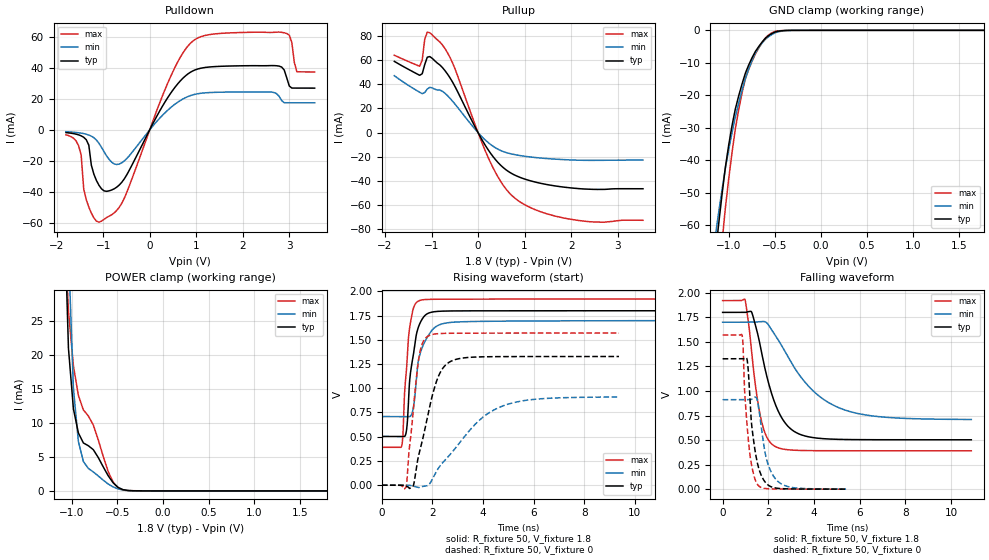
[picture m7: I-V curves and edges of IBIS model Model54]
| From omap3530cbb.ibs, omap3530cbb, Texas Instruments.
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| Model based on original model for CCPV2_7LM
|   Sub model CCPV2_7LM_SN
[model]   Model54
|[Input Load]   PI
|[Output Drive]
|Voltage   1.8V
|Mode   I/O
Model_type   I/O
Polarity   Non-Inverting
Enable   Active-Low
Vinl =  0.63
Vinh =  1.17
Cref =  15.0000pF
Rref =  100.0000M
Vref =  0V
Vmeas =  0.9
C_comp   5.837306p   5.73806p   5.865695p
[Model Spec]
Vinl   0.63   0.595   0.672
Vinh   1.17   1.105   1.248
[Temperature Range]   25   125   -40
[Voltage Range]   1.8   1.7   1.92
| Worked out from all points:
|   slope of the pulldown table from 0 to 0.27 V, typ, clamps not added: 17.9 ohm
|   slope of the pullup table from 0 to 0.27 V, typ, clamps not added: 15.8 ohm
|   GND clamp passes 1 mA (typ) near -0.53 V on its own axis
|   POWER clamp passes 1 mA (typ) near -0.53 V on its own axis
|   rising waveform, R_fixture 50, V_fixture 1.8: 20-80 % time 320ps typ, 436ps min, 234ps max; typ from 0.503 V to 1.8 V
|   rising waveform, R_fixture 50, V_fixture 0: 20-80 % time 728ps typ, 1.88ns min, 370ps max; typ from 0 V to 1.33 V
|   falling waveform, R_fixture 50, V_fixture 1.8: 20-80 % time 928ps typ, 1.98ns min, 523ps max; typ from 1.8 V to 0.503 V
|   falling waveform, R_fixture 50, V_fixture 0: 20-80 % time 361ps typ, 469ps min, 294ps max; typ from 1.33 V to 0 V
[POWER_clamp]
-1.8V     2.373A     2.073A     2.673A
-1.055V   29.19mA    52.52mA    31.79mA
-1.036V   21.01mA    35.61mA    26.49mA
-1.018V   18.03mA    28.77mA    23.8mA
-981.8mV  12.07mA    15.08mA    18.42mA
-927.3mV  8.532mA    7.272mA    14.05mA
-872.7mV  7.067mA    4.332mA    11.93mA
-818.2mV  6.655mA    3.315mA    11.04mA
-763.6mV  6.072mA    2.794mA    9.695mA
-545.5mV  1.18mA     586uA      1.266mA
-381.8mV  61.11uA    52.06uA    52.84uA
1.8V      3.334uA    1.489uA    7.395uA
[Pulldown]
-1.8V     -1.758mA   -1.185mA   -3.17mA
-1.527V   -3.214mA   -1.876mA   -10.31mA
-1.364V   -6.349mA   -2.806mA   -44.88mA
-1.091V   -35.7mA    -8.628mA   -59.51mA
-600mV    -33.78mA   -21.21mA   -47.31mA
436.4mV   23mA       13.98mA    33.48mA
981.8mV   38.72mA    23mA       58.39mA
2.618V    41.46mA    24.35mA    62.82mA
2.891V    38.61mA    17.5mA     62.59mA
3.055V    26.96mA    17.47mA    56.43mA
3.164V    26.94mA    17.45mA    37.42mA
3.545V    26.92mA    17.44mA    37.36mA
[Pullup]
-1.8V     58.82mA    46.97mA    63.88mA
-1.255V   47.3mA     33.32mA    54.75mA
-1.2V     48.59mA    32.13mA    59.92mA
-1.145V   56.22mA    33.1mA     77.08mA
-1.091V   62.26mA    36mA       82.99mA
-818.2mV  55.76mA    35.07mA    74.72mA
-545.5mV  41.54mA    25.83mA    57.35mA
327.3mV   -20.08mA   -11.4mA    -29.4mA
600mV     -30.72mA   -16.43mA   -46.55mA
872.7mV   -36.53mA   -18.79mA   -56.47mA
2.073V    -45.97mA   -22.7mA    -72.08mA
3.545V    -46.38mA   -22.69mA   -72.41mA
[GND_clamp]
-1.8V     -272.3mA   -226.4mA   -345.1mA
-1.145V   -69.37mA   -63.55mA   -89.19mA
-1.109V   -59.79mA   -56.17mA   -76.96mA
-1.073V   -50.76mA   -49.17mA   -65.51mA
-1.036V   -42.26mA   -42.55mA   -54.83mA
-963.6mV  -29.32mA   -31.5mA    -37.62mA
-890.9mV  -20.11mA   -22.34mA   -24.33mA
-818.2mV  -13.14mA   -14.76mA   -14.86mA
-709.1mV  -6.436mA   -6.881mA   -7.201mA
-527.3mV  -895.2uA   -1.203mA   -672.6uA
-309.1mV  -8.844uA   -21.65uA   -7.041uA
1.764V    2.874uA    2.128uA    4.246uA
[Ramp]
dV/dt_f  0.7848143/0.9317531n  0.5993932/1.994104n   0.9269424/0.52629n
dV/dt_r  0.8168281/0.7389269n  0.5610194/1.905523n   0.9665839/0.3758543n
R_load = 50
[Rising Waveform]
R_fixture = 50
V_fixture = 1.8
V_fixture_min = 1.7
V_fixture_max = 1.92
0s        502.9mV    708mV      390.9mV
780ps     502.9mV    708.1mV    401mV
830ps     502.6mV    708.1mV    507.4mV
965ps     550.2mV    707.6mV    1.161V
1.085ns   1.029V     707mV      1.598V
1.255ns   1.36V      812.2mV    1.831V
1.495ns   1.664V     1.34V      1.905V
2.02ns    1.787V     1.609V     1.918V
2.755ns   1.797V     1.68V      1.919V
16.98ns   1.799V     1.698V     1.92V
[Rising Waveform]
R_fixture = 50
V_fixture = 0
V_fixture_min = 0
V_fixture_max = 0
0s        508.5nV    512.5nV    794.3nV
965ps     -9.182mV   106.2uV    -14.86mV
1.245ns   -4.097mV   -9.223mV   776.9mV
1.445ns   295.2mV    -23.32mV   1.28V
1.82ns    725mV      -1.994mV   1.537V
2.28ns    1.148V     191.2mV    1.564V
2.88ns    1.294V     372.6mV    1.568V
3.925ns   1.324V     685.5mV    1.568V
4.95ns    1.326V     832.4mV    1.569V
9.38ns    1.327V     909.3mV    1.569V
[Falling Waveform]
R_fixture = 50
V_fixture = 1.8
V_fixture_min = 1.7
V_fixture_max = 1.92
0s        1.8V       1.7V       1.92V
980ps     1.799V     1.7V       1.929V
1.275ns   1.801V     1.7V       1.384V
1.635ns   1.474V     1.705V     765.3mV
1.905ns   1.178V     1.699V     543.5mV
2.265ns   890.7mV    1.58V      439.5mV
3.16ns    584.3mV    1.231V     396.4mV
4.06ns    522.1mV    980.2mV    392.1mV
5.05ns    507.5mV    833.3mV    391.3mV
10.89ns   503mV      709.7mV    391mV
[Falling Waveform]
R_fixture = 50
V_fixture = 0
V_fixture_min = 0
V_fixture_max = 0
0s        1.327V     911mV      1.569V
855ps     1.327V     911mV      1.565V
970ps     1.332V     910.7mV    969.8mV
1.075ns   1.315V     910.5mV    636.7mV
1.15ns    1.111V     910.6mV    444.1mV
1.275ns   646.5mV    915.3mV    234.9mV
1.545ns   244.8mV    870.8mV    42.13mV
1.915ns   58.21mV    311.1mV    5.74mV
2.39ns    9.618mV    85.65mV    1.965mV
5.405ns   316.4uV    1.705mV    246.8uV
